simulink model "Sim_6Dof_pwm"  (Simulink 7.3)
settings: Solver=ode4  StartTime=0.0  StopTime=80  FixedStep=0.0005  MaxStep=0.0005  RelTol=1e-3
InitFcn:
  | run
StartFcn:
  | run
StopFcn:
  | Pl
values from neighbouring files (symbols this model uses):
  calfa = cos(alfa0*d2r)    [run.m]
  d2r = pi/180    (= 0.0174532925199)    [run.m]
  Kfilt = (wd1^2*wd2^2*wd3^2*wd4^2*wd5^2*wd6^2)/(wn1^2*wn2^2*wn3^2*wn4^2*wn5^2*wn6^2)    (= 0.818930549142)    [run.m]
  klr = lqr(Ap4,Bp4,Q,R)    [run.m]
  kls = lqr(Ap3,Bp3,Q,R)    [run.m]
  r2d = 180/pi    (= 57.2957795131)    [Pl.m]    (also in run.m)
  salfa = sin(alfa0*d2r)    [run.m]
  Thet0 = 43    [run.m]
  V0 = 18640    [run.m]
  wd1 = 29    [run.m]
  wd2 = 37    [run.m]
  wd3 = 40    [run.m]
  wd4 = 48    [run.m]
  wd5 = 63    [run.m]
  wd6 = 68    [run.m]
  wd7 = 34    [run.m]
  wd8 = 19.1    [run.m]
  wlp = 6.6    [run.m]
  wlp2 = 12    [run.m]
  wlpr = 12    [run.m]
  wn1 = 30    [run.m]
  wn2 = 37.9    [run.m]
  wn3 = 40.2    [run.m]
  wn4 = 48.6    [run.m]
  wn5 = 64    [run.m]
  wn6 = 68.6    [run.m]
  wn7 = 34    [run.m]
  wn8 = 19.1    [run.m]
  zd1 = 0.12    [run.m]
  zd2 = 0.12    [run.m]
  zd3 = 0.1    [run.m]
  zd4 = 0.1    [run.m]
  zd5 = 0.1    [run.m]
  zd6 = 0.1    [run.m]
  zd7 = 0.1    [run.m]
  zd8 = 0.1    [run.m]
  zlp = 0.9    [run.m]
  zlp2 = 0.7    [run.m]
  zlpr = 0.7    [run.m]
  zn1 = 0.008    [run.m]
  zn2 = 0.01    [run.m]
  zn3 = 0.01    [run.m]
  zn4 = 0.02    [run.m]
  zn5 = 0.01    [run.m]
  zn6 = 0.01    [run.m]
  zn7 = 0.01    [run.m]
  zn8 = 0.01    [run.m]
undefined symbols (not defined in the file or in its folder): Aai, Aao, Af, Bai, Bao, Bf, Cai, Cao, Cf, Dai, Dao, Df, KSmix, Pos_Thrust3
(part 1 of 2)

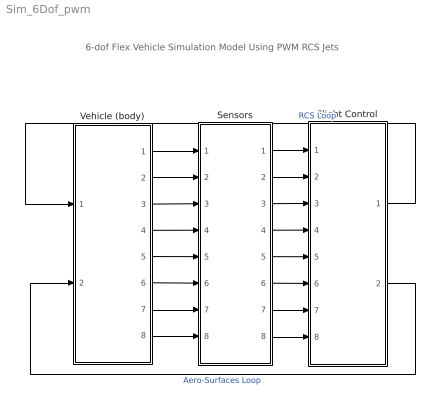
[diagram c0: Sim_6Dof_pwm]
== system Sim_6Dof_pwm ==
  note: 6-dof Flex Vehicle Simulation Model Using PWM RCS Jets
  Flight Control : Subsystem
  Sensors : Subsystem
  Vehicle (body) : Subsystem
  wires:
  Flight Control/2(Aer_pqr) -> Vehicle (body)/2(Aer_pqr)  "Aero-Surfaces Loop"
  Sensors/1(phio) -> Flight Control/1(phi)
  Sensors/2(pbo) -> Flight Control/2(pb)
  Sensors/3(rbo) -> Flight Control/3(rb)
  Sensors/4(beto) -> Flight Control/4(beta)
  Sensors/5(theto) -> Flight Control/5(thet)
  Sensors/6(qo) -> Flight Control/6(q)
  Sensors/7(alfo) -> Flight Control/7(alfa)
  Sensors/8(Nzo) -> Flight Control/8(Nz)
  Vehicle (body)/1(phi) -> Sensors/1(phi)
  Vehicle (body)/2(p) -> Sensors/2(pb)
  Vehicle (body)/3(r) -> Sensors/3(rb)
  Vehicle (body)/4(bet) -> Sensors/4(beta)
  Vehicle (body)/5(thet) -> Sensors/5(thet)
  Vehicle (body)/6(q) -> Sensors/6(q)
  Vehicle (body)/7(alf) -> Sensors/7(alfa)
  Vehicle (body)/8(Nz) -> Sensors/8(Nz)
  Flight Control/1(Jet_pqr) -> Vehicle (body)/1(Jet_PQR_Nz)  "RCS Loop"

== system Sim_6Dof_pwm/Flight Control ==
  note: Flight Control System
  phi : Inport  OutDataType=sfix(16)  OutScaling=2^0
  pb : Inport  Port=2  OutDataType=sfix(16)  OutScaling=2^0
  rb : Inport  Port=3  OutDataType=sfix(16)  OutScaling=2^0
  beta : Inport  Port=4  OutDataType=sfix(16)  OutScaling=2^0
  thet : Inport  Port=5  OutDataType=sfix(16)  OutScaling=2^0
  q : Inport  Port=6  OutDataType=sfix(16)  OutScaling=2^0
  alfa : Inport  Port=7  OutDataType=sfix(16)  OutScaling=2^0
  Nz : Inport  Port=8  OutDataType=sfix(16)  OutScaling=2^0
  1 deg  alfa-comd : Constant  Value=1*d2r  OutDataType=sfix(16)  OutScaling=2^0
  40 deg  phi-cmd : Constant  Value=40*d2r  OutDataType=sfix(16)  OutScaling=2^0
  Body 2 Stabil Transform : Subsystem
  Lateral  Flight Control : Subsystem
  Mix : Subsystem
  Mux1 : Mux  Inputs=[3,1]
  Pitch Flight Control : Subsystem
  Jet_pqr : Outport  OutDataType=sfix(16)  OutScaling=2^0
  Aer_pqr : Outport  Port=2  OutDataType=sfix(16)  OutScaling=2^0
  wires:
  Mux1/1 -> Jet_pqr/1
  Pitch Flight Control/3(Nzfb) -> Mux1/2
  40 deg  phi-cmd/1 -> Lateral  Flight Control/4(phi-cmd)
  1 deg  alfa-comd/1 -> Pitch Flight Control/5(alf-cmd)
  Mix/1(Jet_pqr) -> Mux1/1  "3"
  Nz/1 -> Pitch Flight Control/4(Nz)
  phi/1 -> Body 2 Stabil Transform/1(phi)
  pb/1 -> Body 2 Stabil Transform/2(p_b)
  rb/1 -> Body 2 Stabil Transform/3(r_b)
  Body 2 Stabil Transform/1(p_s) -> Lateral  Flight Control/1(ps)
  Body 2 Stabil Transform/2(r_s) -> Lateral  Flight Control/2(rs)
  alfa/1 -> Pitch Flight Control/3(alf)
  q/1 -> Pitch Flight Control/2(q)
  thet/1 -> Pitch Flight Control/1(thet)
  Mix/2(Aer_pqr) -> Aer_pqr/1  "3"
  beta/1 -> Lateral  Flight Control/3(beta)
  Pitch Flight Control/2(aero_Q) -> Mix/4(Aer_Q)
  Pitch Flight Control/1(rcs_Q) -> Mix/3(Rcs_Q)
  Lateral  Flight Control/2(Aero_PR) -> Mix/2(Aer_PR)
  Lateral  Flight Control/1(Rcs_PR) -> Mix/1(Rcs_PR)

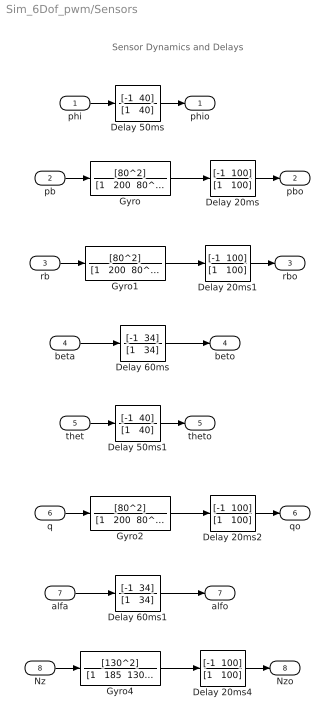
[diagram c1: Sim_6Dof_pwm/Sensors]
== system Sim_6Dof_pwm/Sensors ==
  note: Sensor Dynamics and Delays
  phi : Inport  OutDataType=sfix(16)  OutScaling=2^0
  pb : Inport  Port=2  OutDataType=sfix(16)  OutScaling=2^0
  rb : Inport  Port=3  OutDataType=sfix(16)  OutScaling=2^0
  beta : Inport  Port=4  OutDataType=sfix(16)  OutScaling=2^0
  thet : Inport  Port=5  OutDataType=sfix(16)  OutScaling=2^0
  q : Inport  Port=6  OutDataType=sfix(16)  OutScaling=2^0
  alfa : Inport  Port=7  OutDataType=sfix(16)  OutScaling=2^0
  Nz : Inport  Port=8  OutDataType=sfix(16)  OutScaling=2^0
  Delay 20ms{,1..2,4} (4 alike) : TransferFcn  Numerator="[-1  100]"  Denominator="[1   100]"
  Delay 50ms : TransferFcn  Numerator="[-1  40]"  Denominator="[1   40]"
  Delay 50ms1 : TransferFcn  Numerator="[-1  40]"  Denominator="[1   40]"
  Delay 60ms : TransferFcn  Numerator="[-1  34]"  Denominator="[1   34]"
  Delay 60ms1 : TransferFcn  Numerator="[-1  34]"  Denominator="[1   34]"
  Gyro : TransferFcn  Numerator=[80^2]  Denominator="[1   200  80^2]"
  Gyro1 : TransferFcn  Numerator=[80^2]  Denominator="[1   200  80^2]"
  Gyro2 : TransferFcn  Numerator=[80^2]  Denominator="[1   200  80^2]"
  Gyro4 : TransferFcn  Numerator=[130^2]  Denominator="[1   185  130^2]"
  phio : Outport  OutDataType=sfix(16)  OutScaling=2^0
  pbo : Outport  Port=2  OutDataType=sfix(16)  OutScaling=2^0
  rbo : Outport  Port=3  OutDataType=sfix(16)  OutScaling=2^0
  beto : Outport  Port=4  OutDataType=sfix(16)  OutScaling=2^0
  theto : Outport  Port=5  OutDataType=sfix(16)  OutScaling=2^0
  qo : Outport  Port=6  OutDataType=sfix(16)  OutScaling=2^0
  alfo : Outport  Port=7  OutDataType=sfix(16)  OutScaling=2^0
  Nzo : Outport  Port=8  OutDataType=sfix(16)  OutScaling=2^0
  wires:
  Nz/1 -> Gyro4/1
  Delay 20ms4/1 -> Nzo/1
  Gyro4/1 -> Delay 20ms4/1
  Delay 60ms1/1 -> alfo/1
  alfa/1 -> Delay 60ms1/1
  q/1 -> Gyro2/1
  Delay 20ms2/1 -> qo/1
  Gyro2/1 -> Delay 20ms2/1
  Delay 50ms1/1 -> theto/1
  thet/1 -> Delay 50ms1/1
  Delay 60ms/1 -> beto/1
  beta/1 -> Delay 60ms/1
  rb/1 -> Gyro1/1
  Delay 20ms1/1 -> rbo/1
  Gyro1/1 -> Delay 20ms1/1
  pb/1 -> Gyro/1
  Delay 20ms/1 -> pbo/1
  Delay 50ms/1 -> phio/1
  phi/1 -> Delay 50ms/1
  Gyro/1 -> Delay 20ms/1

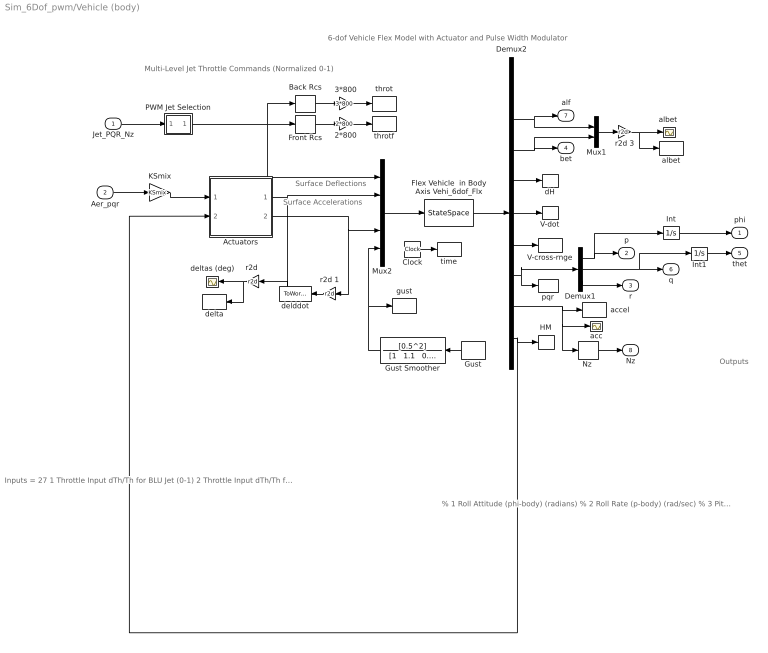
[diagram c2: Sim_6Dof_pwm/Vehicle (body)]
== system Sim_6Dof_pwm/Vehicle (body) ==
  note: Inputs = 27 1 Throttle Input dTh/Th for BLU Jet (0-1) 2 Throttle Input dTh/Th for BRU Jet (0-1) 3 Throttle Input dTh/Th for BLD Jet (0-1) 4 Throttle Input dTh/Th for BRD Jet (0-1) 5 Throttle Input dTh/Th for BL+Y Jet (0-1) 6 Throttle Input dTh/Th for BR-Y Jet (0-1) 7 Throttle Input dTh/Th for FU Jet (0-1) 8 Throttle Input dTh/Th for FLD Jet (0-1) 9 Throttle Input dTh/Th for FRD Jet (0-1) 10 Throttle Input dTh/Th for FL+Y Jet (0-1) 11 Throttle Input dTh/Th for FR-Y Jet (0-1) 12 Left Outbrd Elevon Deflection (radians) 13 Left Inboard Elevon Deflection (radians) 14 Right Inbrd Elevon Deflection (radians) 15 Right Outbrd Elevon Deflection (radians) 16 Vertical Rudder Deflection (radians) 17 Left Outbrd Elevon Velocity (rad/sec) 18 Left Inboard Elevon Velocity (rad/sec) 19 Right Inbrd Elevon Velocity (rad/sec) 20 Right Outbrd Elevon Velocity (rad/sec) 21 Vertical Rudder Velocity (rad/sec) 22 Left Outbrd Elevon Acceleration (rad/s^2) 23 Left Inboard Elevon Acceleration (rad/s^2) 24 Right Inbrd Elevon Acceleration (rad/s^2) 25 Right Outbrd Elevon Acceleration (rad/s^2) 26 Vertical Rudder Acceleration (rad/s^2) 27 Gust Veloc. Azim,Elev=(45, 90) (deg)
  note: Surface Accelerations
  note: Outputs
  note: 6-dof Vehicle Flex Model with Actuator and Pulse Width Modulator
  note: % 1 Roll Attitude (phi-body) (radians) % 2 Roll Rate (p-body) (rad/sec) % 3 Pitch Attitude (thet-bdy) (radians) % 4 Pitch Rate (q-body) (rad/sec) % 5 Yaw Attitude (psi-body) (radians) % 6 Yaw Rate (r-body) (rad/sec) % 7 Angle of attack, alfa, (radians) % 8 Angle of sideslip, beta, (radian) % 9 Change in Altitude, delta-h, (feet) % 10 Forward Acceleration (V-dot) (ft/sec) % 11 Cross Range Velocity (Vcr) (ft/sec) % 12 Rate-Gyro # 1, Roll Rate (Body) (rad/sec) % 13 Rate-Gyro # 2, Pitch Rate (Body) (rad/sec) % 14 Rate-Gyro # 3, Yaw Rate (Body) (rad/sec) % 15 Accelerom # 1, (along X), (ft/sec^2) Translat. Acceler % 16 Accelerom # 2, (along Y), (ft/sec^2) Translat. Acceler % 17 Accelerom # 3, (along Z), (ft/sec^2) Translat. Acceler % 18 Hinge Moment for Aero Surface # 1, (ft-lb) % 19 Hinge Moment for Aero Surface # 2, (ft-lb) % 20 Hinge Moment for Aero Surface # 3, (ft-lb) % 21 Hinge Moment for Aero Surface # 4, (ft-lb) % 22 Hinge Moment for Aero Surface # 5, (ft-lb)
  note: Multi-Level Jet Throttle Commands (Normalized 0-1)
  note: Surface Deflections
  Jet_PQR_Nz : Inport  OutDataType=sfix(16)  OutScaling=2^0
  Aer_pqr : Inport  Port=2  OutDataType=sfix(16)  OutScaling=2^0
  2*800 : Gain  Gain=2*800  ParameterDataType=sfix(16)  ParameterScaling=2^0  OutDataType=sfix(16)  OutScaling=2^0
  3*800 : Gain  Gain=3*800  ParameterDataType=sfix(16)  ParameterScaling=2^0  OutDataType=sfix(16)  OutScaling=2^0
  Actuators : Subsystem
  Back Rcs : Selector  InputPortWidth=11  IndexOptions=Index vector (dialog)  Indices=[1:6]  OutputSizes=1
  Clock : Clock
  Demux1 : Demux  Outputs=3
  Demux2 : Demux  Outputs="[6 1 1 1 1 1 3  3  5]"
  Flex Vehicle  in Body Axis Vehi_6dof_Flx : StateSpace  A=Af  B=Bf  C=Cf  D=Df
  Front Rcs : Selector  InputPortWidth=11  IndexOptions=Index vector (dialog)  Indices=[7:11]  OutputSizes=1
  Gust : DiscretePulseGenerator  PulseType=Time based  Amplitude=50  Period=500  PulseWidth=10  PhaseDelay=0  SampleTime=1
  Gust Smoother : TransferFcn  Numerator=[0.5^2]  Denominator="[1   1.1   0.5^2]"
  HM : ToWorkspace  VariableName=HM  SampleTime=-1  SaveFormat=Array
  Int : Integrator
  Int1 : Integrator
  KSmix : Gain  Gain=KSmix  Multiplication=Matrix(K*u)  ParameterDataType=sfix(16)  ParameterScaling=2^0  OutDataType=sfix(16)  OutScaling=2^0
  Mux1 : Mux  Inputs=2
  Mux2 : Mux  Inputs=[11, 5,5,5, 1]
  "Nz " : Selector  InputPortWidth=3  IndexOptions=Index vector (dialog)  Indices=[3]  OutputSizes=1
  PWM Jet Selection : Subsystem
  V-cross-rnge : ToWorkspace  VariableName=Vxrng  SampleTime=-1  SaveFormat=Array
  V-dot : ToWorkspace  VariableName=dV  SampleTime=-1  SaveFormat=Array
  acc : Scope
  accel : ToWorkspace  VariableName=accel  SampleTime=-1  SaveFormat=Array
  albet : ToWorkspace  VariableName=albet  SampleTime=-1  SaveFormat=Array
  "albet " : Scope
  dH : ToWorkspace  VariableName=dH  SampleTime=-1  SaveFormat=Array
  delddot : ToWorkspace  VariableName=delddot  SampleTime=-1  SaveFormat=Array
  delta : ToWorkspace  VariableName=delta  SampleTime=-1  SaveFormat=Array
  deltas (deg) : Scope
  gust : ToWorkspace  VariableName=gust  SampleTime=-1  SaveFormat=Array
  pqr : ToWorkspace  VariableName=pqr  SampleTime=-1  SaveFormat=Array
  "r2d " : Gain  Gain=r2d  ParameterDataType=sfix(16)  ParameterScaling=2^0  OutDataType=sfix(16)  OutScaling=2^0
  r2d 1 : Gain  Gain=r2d  ParameterDataType=sfix(16)  ParameterScaling=2^0  OutDataType=sfix(16)  OutScaling=2^0
  r2d 3 : Gain  Gain=r2d  ParameterDataType=sfix(16)  ParameterScaling=2^0  OutDataType=sfix(16)  OutScaling=2^0
  throt : ToWorkspace  VariableName=throtb  SampleTime=-1  SaveFormat=Array
  throtf : ToWorkspace  VariableName=throtf  SampleTime=-1  SaveFormat=Array
  time : ToWorkspace  VariableName=time  SampleTime=-1  SaveFormat=Array
  phi : Outport  OutDataType=sfix(16)  OutScaling=2^0
  p : Outport  Port=2  OutDataType=sfix(16)  OutScaling=2^0
  r : Outport  Port=3  OutDataType=sfix(16)  OutScaling=2^0
  bet : Outport  Port=4  OutDataType=sfix(16)  OutScaling=2^0
  thet : Outport  Port=5  OutDataType=sfix(16)  OutScaling=2^0
  q : Outport  Port=6  OutDataType=sfix(16)  OutScaling=2^0
  alf : Outport  Port=7  OutDataType=sfix(16)  OutScaling=2^0
  Nz : Outport  Port=8  OutDataType=sfix(16)  OutScaling=2^0
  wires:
  Actuators/2(delddot) -> Mux2/4, r2d 1/1
  KSmix/1 -> Actuators/1(delcom)
  Actuators/1(delta) -> Mux2/2, "r2d "/1
  Jet_PQR_Nz/1 -> PWM Jet Selection/1(In)
  Aer_pqr/1 -> KSmix/1
  Mux2/1 -> Flex Vehicle  in Body Axis Vehi_6dof_Flx/1
  PWM Jet Selection/1(Ot) -> Mux2/1, Back Rcs/1, Front Rcs/1
  "r2d "/1 -> deltas (deg)/1, delta/1
  r2d 1/1 -> delddot/1
  Gust/1 -> Gust Smoother/1
  Clock/1 -> time/1
  Gust Smoother/1 -> Mux2/5, gust/1
  r2d 3/1 -> "albet "/1, albet/1
  Mux1/1 -> r2d 3/1
  Flex Vehicle  in Body Axis Vehi_6dof_Flx/1 -> Demux2/1
  Demux2/9 -> HM/1, Actuators/2(HM)
  Demux2/8 -> accel/1, acc/1, "Nz "/1
  "Nz "/1 -> Nz/1
  Demux2/7 -> pqr/1, Demux1/1
  Demux1/1 -> p/1, Int/1
  Demux1/2 -> q/1, Int1/1
  Demux1/3 -> r/1
  Demux2/6 -> V-cross-rnge/1
  Demux2/5 -> V-dot/1
  Demux2/4 -> dH/1
  Demux2/2 -> alf/1, Mux1/1
  Demux2/3 -> bet/1, Mux1/2
  Int1/1 -> thet/1
  Int/1 -> phi/1
  Back Rcs/1 -> 3*800/1
  Front Rcs/1 -> 2*800/1
  3*800/1 -> throt/1
  2*800/1 -> throtf/1

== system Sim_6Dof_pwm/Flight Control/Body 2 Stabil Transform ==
  note: Body to Stability Axes Transformation
  phi : Inport  OutDataType=sfix(16)  OutScaling=2^0
  p_b : Inport  Port=2  OutDataType=sfix(16)  OutScaling=2^0
  r_b : Inport  Port=3  OutDataType=sfix(16)  OutScaling=2^0
  Mux1 : Mux  Inputs=2
  Sum1 : Sum  Inputs=+|+  OutDataType=sfix(16)  OutScaling=2^0
  Sum2 : Sum  Inputs=+|-  OutDataType=sfix(16)  OutScaling=2^0
  Sum3 : Sum  Inputs=|++  OutDataType=sfix(16)  OutScaling=2^0
  Sum4 : Sum  Inputs=|+-  OutDataType=sfix(16)  OutScaling=2^0
  calfa : Gain  Gain=calfa  ParameterDataType=sfix(16)  ParameterScaling=2^0  OutDataType=sfix(16)  OutScaling=2^0
  "calfa " : Gain  Gain=calfa  ParameterDataType=sfix(16)  ParameterScaling=2^0  OutDataType=sfix(16)  OutScaling=2^0
  g cos(Thet0) /V0 : Gain  Gain=32.2*cos(Thet0*d2r)/V0  ParameterDataType=sfix(16)  ParameterScaling=2^0  OutDataType=sfix(16)  OutScaling=2^0
  g sin(Thet0) /V0 : Gain  Gain=32.2*sin(Thet0*d2r)/V0  ParameterDataType=sfix(16)  ParameterScaling=2^0  OutDataType=sfix(16)  OutScaling=2^0
  pr_stabil : ToWorkspace  VariableName=pr_st  SampleTime=-1  SaveFormat=Array
  salfa : Gain  Gain=salfa  ParameterDataType=sfix(16)  ParameterScaling=2^0  OutDataType=sfix(16)  OutScaling=2^0
  "salfa " : Gain  Gain=salfa  ParameterDataType=sfix(16)  ParameterScaling=2^0  OutDataType=sfix(16)  OutScaling=2^0
  p_s : Outport  OutDataType=sfix(16)  OutScaling=2^0
  r_s : Outport  Port=2  OutDataType=sfix(16)  OutScaling=2^0
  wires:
  Mux1/1 -> pr_stabil/1
  "salfa "/1 -> Sum2/2
  "calfa "/1 -> Sum2/1
  salfa/1 -> Sum1/2
  calfa/1 -> Sum1/1
  Sum3/1 -> calfa/1, "salfa "/1
  Sum4/1 -> salfa/1, "calfa "/1
  phi/1 -> g sin(Thet0) /V0/1, g cos(Thet0) /V0/1
  g sin(Thet0) /V0/1 -> Sum4/2
  g cos(Thet0) /V0/1 -> Sum3/2
  r_b/1 -> Sum4/1
  p_b/1 -> Sum3/1
  Sum2/1 -> Mux1/2, r_s/1
  Sum1/1 -> Mux1/1, p_s/1

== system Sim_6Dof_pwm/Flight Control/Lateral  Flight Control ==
  note: Lateral Flight Control System
  ps : Inport  OutDataType=sfix(16)  OutScaling=2^0
  rs : Inport  Port=2  OutDataType=sfix(16)  OutScaling=2^0
  beta : Inport  Port=3  OutDataType=sfix(16)  OutScaling=2^0
  phi-cmd : Inport  Port=4  OutDataType=sfix(16)  OutScaling=2^0
  5 state Aero feedback : Gain  Gain=-kls  Multiplication=Matrix(K*u)  ParameterDataType=sfix(16)  ParameterScaling=2^0  OutDataType=sfix(16)  OutScaling=2^0
  5 state RCS feedback : Gain  Gain=-klr  Multiplication=Matrix(K*u)  ParameterDataType=sfix(16)  ParameterScaling=2^0  OutDataType=sfix(16)  OutScaling=2^0
  Filters : Subsystem
  Int : Integrator
  "Int " : Integrator
  Mux3 : Mux  Inputs=5
  RCS Filters : Subsystem
  Sum : Sum  Inputs=|+-  OutDataType=sfix(16)  OutScaling=2^0
  phi : Scope
  phi-stabil : ToWorkspace  VariableName=phi_st  SampleTime=-1  SaveFormat=Array
  r2d : Gain  Gain=r2d  ParameterDataType=sfix(16)  ParameterScaling=2^0  OutDataType=sfix(16)  OutScaling=2^0
  Rcs_PR : Outport  OutDataType=sfix(16)  OutScaling=2^0
  Aero_PR : Outport  Port=2  OutDataType=sfix(16)  OutScaling=2^0
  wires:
  RCS Filters/1(Ou) -> Rcs_PR/1
  Filters/1(Ou) -> Aero_PR/1
  r2d/1 -> phi-stabil/1, phi/1
  phi-cmd/1 -> Sum/2
  5 state Aero feedback/1 -> Filters/1(In)  "aero(P,R)"
  5 state RCS feedback/1 -> RCS Filters/1(In)  "rcs(P,R)"
  rs/1 -> Mux3/2
  Mux3/1 -> 5 state RCS feedback/1, 5 state Aero feedback/1
  ps/1 -> Mux3/1, "Int "/1
  beta/1 -> Mux3/3, Int/1
  Int/1 -> Mux3/5  "beti"
  Sum/1 -> Mux3/4
  "Int "/1 -> r2d/1, Sum/1  "pint"

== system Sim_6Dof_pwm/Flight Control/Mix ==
  Rcs_PR : Inport  OutDataType=sfix(16)  OutScaling=2^0
  Aer_PR : Inport  Port=2  OutDataType=sfix(16)  OutScaling=2^0
  Rcs_Q : Inport  Port=3  OutDataType=sfix(16)  OutScaling=2^0
  Aer_Q : Inport  Port=4  OutDataType=sfix(16)  OutScaling=2^0
  Demux1 : Demux  Outputs=2
  Demux2 : Demux  Outputs=2
  Mux1 : Mux  Inputs=3
  Mux2 : Mux  Inputs=3
  Jet_pqr : Outport  OutDataType=sfix(16)  OutScaling=2^0
  Aer_pqr : Outport  Port=2  OutDataType=sfix(16)  OutScaling=2^0
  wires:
  Rcs_Q/1 -> Mux1/2
  Mux2/1 -> Aer_pqr/1
  Aer_Q/1 -> Mux2/2
  Aer_PR/1 -> Demux2/1
  Rcs_PR/1 -> Demux1/1
  Mux1/1 -> Jet_pqr/1
  Demux2/2 -> Mux2/3
  Demux2/1 -> Mux2/1
  Demux1/2 -> Mux1/3
  Demux1/1 -> Mux1/1

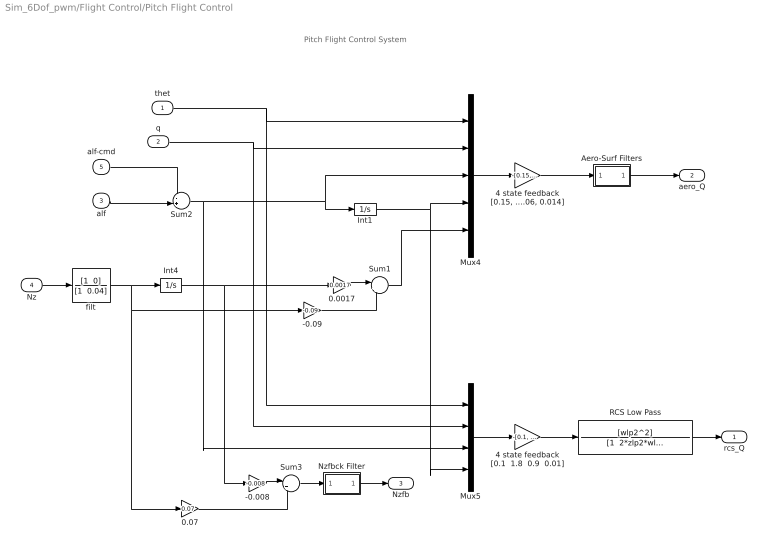
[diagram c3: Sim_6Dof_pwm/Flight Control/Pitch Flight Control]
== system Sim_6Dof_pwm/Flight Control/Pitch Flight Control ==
  note: Pitch Flight Control System
  thet : Inport  OutDataType=sfix(16)  OutScaling=2^0
  q : Inport  Port=2  OutDataType=sfix(16)  OutScaling=2^0
  alf : Inport  Port=3  OutDataType=sfix(16)  OutScaling=2^0
  Nz : Inport  Port=4  OutDataType=sfix(16)  OutScaling=2^0
  alf-cmd : Inport  Port=5  OutDataType=sfix(16)  OutScaling=2^0
  -0.008 : Gain  Gain=-0.008  ParameterDataType=sfix(16)  ParameterScaling=2^0  OutDataType=sfix(16)  OutScaling=2^0
  -0.09 : Gain  Gain=-0.09  ParameterDataType=sfix(16)  ParameterScaling=2^0  OutDataType=sfix(16)  OutScaling=2^0
  0.0017 : Gain  Gain=0.0017  ParameterDataType=sfix(16)  ParameterScaling=2^0  OutDataType=sfix(16)  OutScaling=2^0
  0.07 : Gain  Gain=0.07  ParameterDataType=sfix(16)  ParameterScaling=2^0  OutDataType=sfix(16)  OutScaling=2^0
  4 state feedback [0.1  1.8  0.9  0.01] : Gain  Gain="-[0.1,   1.8,   0.9,    0.01]"  Multiplication=Matrix(K*u)  ParameterDataType=sfix(16)  ParameterScaling=2^0  OutDataType=sfix(16)  OutScaling=2^0
  "4 state feedback [0.15, 2, 0.9, 0.06, 0.014]" : Gain  Gain="-[0.15,   2,   0.9,    0.06,   0.015]"  Multiplication=Matrix(K*u)  ParameterDataType=sfix(16)  ParameterScaling=2^0  OutDataType=sfix(16)  OutScaling=2^0
  Aero-Surf Filters : Subsystem
  Int1 : Integrator
  Int4 : Integrator
  Mux4 : Mux  Inputs=5
  Mux5 : Mux
  Nzfbck Filter : Subsystem
  RCS Low Pass : TransferFcn  Numerator=[wlp2^2]  Denominator="[1  2*zlp2*wlp2  wlp2^2]"
  Sum1 : Sum  Inputs=|++  OutDataType=sfix(16)  OutScaling=2^0
  Sum2 : Sum  Inputs=-+|  OutDataType=sfix(16)  OutScaling=2^0
  Sum3 : Sum  Inputs=|++  OutDataType=sfix(16)  OutScaling=2^0
  filt : TransferFcn  Numerator="[1  0]"  Denominator="[1  0.04]"
  rcs_Q : Outport  OutDataType=sfix(16)  OutScaling=2^0
  aero_Q : Outport  Port=2  OutDataType=sfix(16)  OutScaling=2^0
  Nzfb : Outport  Port=3  OutDataType=sfix(16)  OutScaling=2^0
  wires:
  RCS Low Pass/1 -> rcs_Q/1
  Sum3/1 -> Nzfbck Filter/1(in)
  Int1/1 -> Mux4/4, Mux5/4
  Sum2/1 -> Int1/1, Mux4/3, Mux5/3
  thet/1 -> Mux4/1, Mux5/1
  q/1 -> Mux4/2, Mux5/2
  0.0017/1 -> Sum1/1
  -0.09/1 -> Sum1/2
  Nz/1 -> filt/1
  Sum1/1 -> Mux4/5
  Mux4/1 -> "4 state feedback [0.15, 2, 0.9, 0.06, 0.014]"/1
  "4 state feedback [0.15, 2, 0.9, 0.06, 0.014]"/1 -> Aero-Surf Filters/1(in)
  Mux5/1 -> 4 state feedback [0.1  1.8  0.9  0.01]/1
  4 state feedback [0.1  1.8  0.9  0.01]/1 -> RCS Low Pass/1
  0.07/1 -> Sum3/2
  -0.008/1 -> Sum3/1
  Int4/1 -> 0.0017/1, -0.008/1
  filt/1 -> Int4/1, -0.09/1, 0.07/1
  alf/1 -> Sum2/2
  alf-cmd/1 -> Sum2/1
  Nzfbck Filter/1(ot) -> Nzfb/1
  Aero-Surf Filters/1(ot) -> aero_Q/1

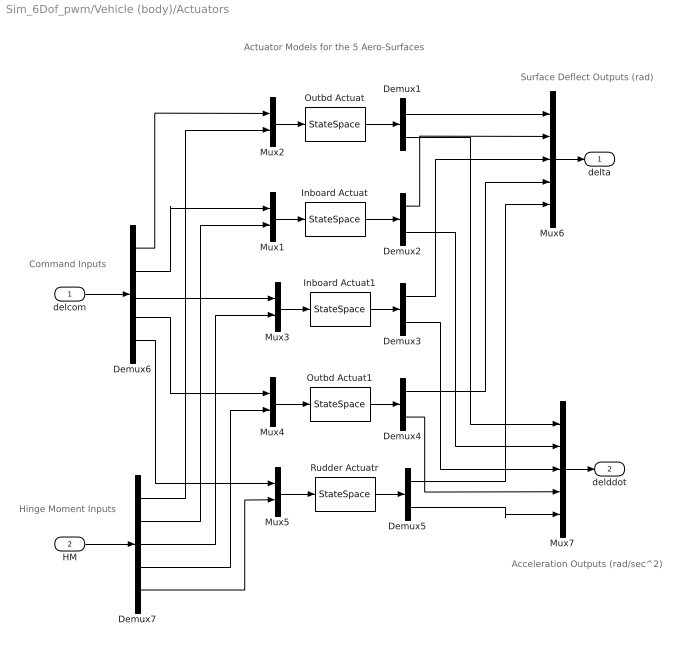
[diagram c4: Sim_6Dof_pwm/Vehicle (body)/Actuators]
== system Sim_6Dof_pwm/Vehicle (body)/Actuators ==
  note: Command Inputs
  note: Hinge Moment Inputs
  note: Actuator Models for the 5 Aero-Surfaces
  note: Acceleration Outputs (rad/sec^2)
  note: Surface Deflect Outputs (rad)
  delcom : Inport  OutDataType=sfix(16)  OutScaling=2^0
  HM : Inport  Port=2  OutDataType=sfix(16)  OutScaling=2^0
  Demux{1..5} (5 alike) : Demux  Outputs=3
  Demux6 : Demux  Outputs=5
  Demux7 : Demux  Outputs=5
  Inboard Actuat : StateSpace  A=Aai  B=Bai  C=Cai  D=Dai
  Inboard Actuat1 : StateSpace  A=Aai  B=Bai  C=Cai  D=Dai
  Mux{1..5} (5 alike) : Mux  Inputs=2
  Mux6 : Mux  Inputs=5
  Mux7 : Mux  Inputs=5
  Outbd Actuat : StateSpace  A=Aao  B=Bao  C=Cao  D=Dao
  Outbd Actuat1 : StateSpace  A=Aao  B=Bao  C=Cao  D=Dao
  Rudder Actuatr : StateSpace  A=Aai  B=Bai  C=Cai  D=Dai
  delta : Outport  OutDataType=sfix(16)  OutScaling=2^0
  delddot : Outport  Port=2  OutDataType=sfix(16)  OutScaling=2^0
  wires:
  Mux6/1 -> delta/1
  Mux7/1 -> delddot/1
  Mux1/1 -> Inboard Actuat/1
  Mux2/1 -> Outbd Actuat/1
  Mux3/1 -> Inboard Actuat1/1
  Mux4/1 -> Outbd Actuat1/1
  Mux5/1 -> Rudder Actuatr/1
  Outbd Actuat/1 -> Demux1/1
  Inboard Actuat/1 -> Demux2/1
  Inboard Actuat1/1 -> Demux3/1
  Outbd Actuat1/1 -> Demux4/1
  Rudder Actuatr/1 -> Demux5/1
  delcom/1 -> Demux6/1
  Demux6/1 -> Mux2/1
  Demux6/2 -> Mux1/1
  Demux6/3 -> Mux3/1
  Demux6/4 -> Mux4/1
  Demux6/5 -> Mux5/1
  Demux5/3 -> Mux7/5
  Demux4/3 -> Mux7/4
  Demux3/3 -> Mux7/3
  Demux2/3 -> Mux7/2
  Demux1/3 -> Mux7/1
  Demux1/1 -> Mux6/1
  Demux2/1 -> Mux6/2
  Demux3/1 -> Mux6/3
  Demux4/1 -> Mux6/4
  Demux5/1 -> Mux6/5
  Demux7/1 -> Mux2/2
  Demux7/2 -> Mux1/2
  Demux7/3 -> Mux3/2
  Demux7/4 -> Mux4/2
  Demux7/5 -> Mux5/2
  HM/1 -> Demux7/1

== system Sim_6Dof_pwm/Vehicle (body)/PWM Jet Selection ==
  note: Jet Selection Logic
  In : Inport  OutDataType=sfix(16)  OutScaling=2^0
  Demux2 : Demux  Outputs="[3  3  3  3  3  3  2  2  2  2  2  1]"
  Mem : Memory
  Mix Logic +ve thrusts : MATLABFcn  MATLABFcn=Pos_Thrust3(u(1:4) )  OutputDimensions=6*3 + 5*2 + 1  OutputSignalType=real
  Mux1 : Mux  Inputs=11
  PW Modulators : Subsystem
  error : Scope
  error-magn : ToWorkspace  VariableName=erm  SampleTime=-1  SaveFormat=Array
  Ot : Outport  OutDataType=sfix(16)  OutScaling=2^0
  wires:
  Demux2/12 -> error-magn/1, error/1
  Mix Logic +ve thrusts/1 -> Demux2/1
  PW Modulators/11(O10) -> Mux1/11
  PW Modulators/10(O9) -> Mux1/10
  PW Modulators/9(O8) -> Mux1/9
  PW Modulators/8(O7) -> Mux1/8
  PW Modulators/7(O6) -> Mux1/7
  PW Modulators/6(O5) -> Mux1/6
  PW Modulators/5(O4) -> Mux1/5
  PW Modulators/4(O3) -> Mux1/4
  PW Modulators/3(O2) -> Mux1/3
  PW Modulators/2(O1) -> Mux1/2
  PW Modulators/1(O) -> Mux1/1
  Demux2/11 -> PW Modulators/11(In10)
  Demux2/10 -> PW Modulators/10(In9)
  Demux2/9 -> PW Modulators/9(In8)
  Demux2/8 -> PW Modulators/8(In7)
  Demux2/7 -> PW Modulators/7(In6)
  Demux2/6 -> PW Modulators/6(In5)
  Demux2/5 -> PW Modulators/5(In4)
  Demux2/4 -> PW Modulators/4(In3)
  Demux2/3 -> PW Modulators/3(In2)
  Demux2/2 -> PW Modulators/2(In1)
  Demux2/1 -> PW Modulators/1(In)
  Mem/1 -> Mix Logic +ve thrusts/1
  Mux1/1 -> Ot/1
  In/1 -> Mem/1

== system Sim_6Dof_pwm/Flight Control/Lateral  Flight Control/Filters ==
  In : Inport  OutDataType=sfix(16)  OutScaling=2^0
  19.1 r/s Notch1 : TransferFcn  Numerator="[1  2*zn8*wn8  wn8^2]"  Denominator="[1  2*zd8*wd8  wd8^2]"
  34 r/s Notch : TransferFcn  Numerator="[1  2*zn7*wn7  wn7^2]"  Denominator="[1  2*zd7*wd7  wd7^2]"
  Demux1 : Demux  Outputs=2
  Mux1 : Mux  Inputs=2
  Roll Low Pass : TransferFcn  Numerator=[wlp^2]  Denominator="[1  1.3*wlp  wlp^2]"
  Yaw Low Pass : TransferFcn  Numerator=[wlp^2]  Denominator="[1  1.3*wlp  wlp^2]"
  Ou : Outport  OutDataType=sfix(16)  OutScaling=2^0
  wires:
  19.1 r/s Notch1/1 -> Yaw Low Pass/1
  34 r/s Notch/1 -> Roll Low Pass/1
  Yaw Low Pass/1 -> Mux1/2
  Demux1/2 -> 19.1 r/s Notch1/1
  Roll Low Pass/1 -> Mux1/1
  Mux1/1 -> Ou/1
  Demux1/1 -> 34 r/s Notch/1
  In/1 -> Demux1/1

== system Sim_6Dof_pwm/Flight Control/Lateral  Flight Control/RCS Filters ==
  In : Inport  OutDataType=sfix(16)  OutScaling=2^0
  Demux1 : Demux  Outputs=2
  Mux1 : Mux  Inputs=2
  RCS Low Pass : TransferFcn  Numerator=[wlpr^2]  Denominator="[1  2*zlpr*wlpr  wlpr^2]"
  RCS Low Pass1 : TransferFcn  Numerator=[wlpr^2]  Denominator="[1  2*zlpr*wlpr  wlpr^2]"
  Ou : Outport  OutDataType=sfix(16)  OutScaling=2^0
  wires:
  RCS Low Pass1/1 -> Mux1/2
  RCS Low Pass/1 -> Mux1/1
  Demux1/2 -> RCS Low Pass1/1
  Mux1/1 -> Ou/1
  Demux1/1 -> RCS Low Pass/1
  In/1 -> Demux1/1

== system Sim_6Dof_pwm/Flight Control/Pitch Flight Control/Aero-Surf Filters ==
  note: Pitch Flexibility Filters
  in : Inport  OutDataType=sfix(16)  OutScaling=2^0
  30 r/s Notch : TransferFcn  Numerator="[1  2*zn1*wn1  wn1^2]"  Denominator="[1  2*zd1*wd1  wd1^2]"
  34 r/s Notch1 : TransferFcn  Numerator="[1  2*zn7*wn7  wn7^2]"  Denominator="[1  2*zd7*wd7  wd7^2]"
  37.9 r/s Notch : TransferFcn  Numerator="[1  2*zn2*wn2  wn2^2]"  Denominator="[1  2*zd2*wd2  wd2^2]"
  40.2 r/s Notch : TransferFcn  Numerator="[1  2*zn3*wn3  wn3^2]"  Denominator="[1  2*zd3*wd3  wd3^2]"
  48.6 r/s Notch : TransferFcn  Numerator="[1  2*zn4*wn4  wn4^2]"  Denominator="[1  2*zd4*wd4  wd4^2]"
  64 r/s Notch : TransferFcn  Numerator="[1  2*zn5*wn5  wn5^2]"  Denominator="[1  2*zd5*wd5  wd5^2]"
  68 r/s Notch : TransferFcn  Numerator="[1  2*zn6*wn6  wn6^2]"  Denominator="[1  2*zd6*wd6  wd6^2]"
  9 r/s Notch : TransferFcn  Numerator="[1  0.04*9  8.5^2]"  Denominator="[1  0.2*9  8.5^2]"
  Kfilt : Gain  Gain=Kfilt  ParameterDataType=sfix(16)  ParameterScaling=2^0  OutDataType=sfix(16)  OutScaling=2^0
  Low Pass : TransferFcn  Numerator=[wlp^2]  Denominator="[1  2*zlp*wlp  wlp^2]"
  ot : Outport  OutDataType=sfix(16)  OutScaling=2^0
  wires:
  in/1 -> 30 r/s Notch/1
  30 r/s Notch/1 -> 37.9 r/s Notch/1
  37.9 r/s Notch/1 -> 40.2 r/s Notch/1
  40.2 r/s Notch/1 -> 48.6 r/s Notch/1
  Kfilt/1 -> ot/1
  68 r/s Notch/1 -> 34 r/s Notch1/1
  Low Pass/1 -> Kfilt/1
  48.6 r/s Notch/1 -> 64 r/s Notch/1
  64 r/s Notch/1 -> 68 r/s Notch/1
  9 r/s Notch/1 -> Low Pass/1
  34 r/s Notch1/1 -> 9 r/s Notch/1

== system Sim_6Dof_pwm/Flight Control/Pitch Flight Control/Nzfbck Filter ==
  note: Nz feedback Filters
  in : Inport  OutDataType=sfix(16)  OutScaling=2^0
  30 r/s Notch : TransferFcn  Numerator="[1  2*zn1*wn1  wn1^2]"  Denominator="[1  2*zd1*wd1  wd1^2]"
  RCS Low Pass1 : TransferFcn  Numerator=[wlp2^2]  Denominator="[1  2*zlp2*wlp2  wlp2^2]"
  ot : Outport  OutDataType=sfix(16)  OutScaling=2^0
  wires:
  in/1 -> 30 r/s Notch/1
  30 r/s Notch/1 -> RCS Low Pass1/1
  RCS Low Pass1/1 -> ot/1

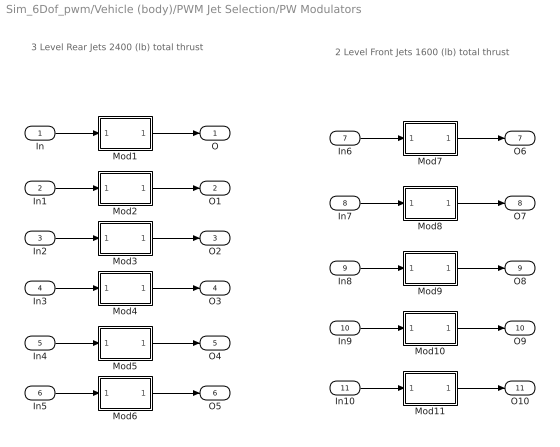
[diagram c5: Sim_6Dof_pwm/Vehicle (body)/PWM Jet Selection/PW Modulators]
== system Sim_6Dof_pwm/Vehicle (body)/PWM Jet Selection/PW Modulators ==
  note: 2 Level Front Jets 1600 (lb) total thrust
  note: 3 Level Rear Jets 2400 (lb) total thrust
  In : Inport  OutDataType=sfix(16)  OutScaling=2^0
  In1 : Inport  Port=2  OutDataType=sfix(16)  OutScaling=2^0
  In2 : Inport  Port=3  OutDataType=sfix(16)  OutScaling=2^0
  In3 : Inport  Port=4  OutDataType=sfix(16)  OutScaling=2^0
  In4 : Inport  Port=5  OutDataType=sfix(16)  OutScaling=2^0
  In5 : Inport  Port=6  OutDataType=sfix(16)  OutScaling=2^0
  In6 : Inport  Port=7  OutDataType=sfix(16)  OutScaling=2^0
  In7 : Inport  Port=8  OutDataType=sfix(16)  OutScaling=2^0
  In8 : Inport  Port=9  OutDataType=sfix(16)  OutScaling=2^0
  In9 : Inport  Port=10  OutDataType=sfix(16)  OutScaling=2^0
  In10 : Inport  Port=11  OutDataType=sfix(16)  OutScaling=2^0
  Mod1 : Subsystem
  Mod10 : Subsystem
  Mod11 : Subsystem
  Mod2 : Subsystem
  Mod3 : Subsystem
  Mod4 : Subsystem
  Mod5 : Subsystem
  Mod6 : Subsystem
  Mod7 : Subsystem
  Mod8 : Subsystem
  Mod9 : Subsystem
  O : Outport  OutDataType=sfix(16)  OutScaling=2^0
  O1 : Outport  Port=2  OutDataType=sfix(16)  OutScaling=2^0
  O2 : Outport  Port=3  OutDataType=sfix(16)  OutScaling=2^0
  O3 : Outport  Port=4  OutDataType=sfix(16)  OutScaling=2^0
  O4 : Outport  Port=5  OutDataType=sfix(16)  OutScaling=2^0
  O5 : Outport  Port=6  OutDataType=sfix(16)  OutScaling=2^0
  O6 : Outport  Port=7  OutDataType=sfix(16)  OutScaling=2^0
  O7 : Outport  Port=8  OutDataType=sfix(16)  OutScaling=2^0
  O8 : Outport  Port=9  OutDataType=sfix(16)  OutScaling=2^0
  O9 : Outport  Port=10  OutDataType=sfix(16)  OutScaling=2^0
  O10 : Outport  Port=11  OutDataType=sfix(16)  OutScaling=2^0
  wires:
  In10/1 -> Mod11/1(In1)
  Mod11/1(O1) -> O10/1
  In9/1 -> Mod10/1(In1)
  Mod10/1(O1) -> O9/1
  In8/1 -> Mod9/1(In1)
  Mod9/1(O1) -> O8/1
  In7/1 -> Mod8/1(In1)
  Mod8/1(O1) -> O7/1
  In6/1 -> Mod7/1(In1)
  Mod7/1(O1) -> O6/1
  In5/1 -> Mod6/1(In1)
  Mod6/1(O1) -> O5/1
  In4/1 -> Mod5/1(In1)
  Mod5/1(O1) -> O4/1
  In3/1 -> Mod4/1(In1)
  Mod4/1(O1) -> O3/1
  In2/1 -> Mod3/1(In1)
  Mod3/1(O1) -> O2/1
  In1/1 -> Mod2/1(In1)
  Mod2/1(O1) -> O1/1
  In/1 -> Mod1/1(In1)
  Mod1/1(O1) -> O/1

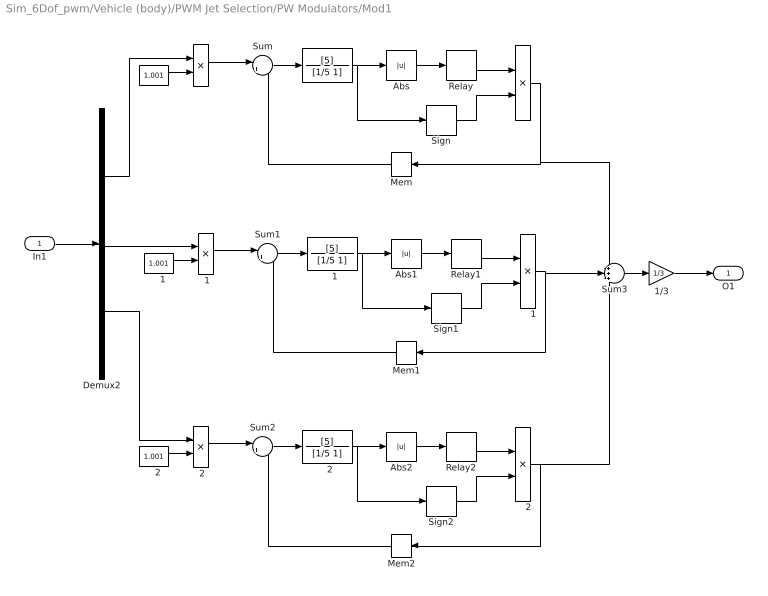
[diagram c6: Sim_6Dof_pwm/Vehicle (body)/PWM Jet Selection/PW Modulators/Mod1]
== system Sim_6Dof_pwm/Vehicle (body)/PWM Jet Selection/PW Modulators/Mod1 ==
  In1 : Inport  OutDataType=sfix(16)  OutScaling=2^0
  " " : Product  OutDataType=sfix(16)  OutScaling=2^0
  "  " : TransferFcn  Numerator=[5]  Denominator=[1/5 1]
  "   " : Constant  Value=1.001  OutDataType=sfix(16)  OutScaling=2^0
  "    " : Product  OutDataType=sfix(16)  OutScaling=2^0
  "    1" : Product  OutDataType=sfix(16)  OutScaling=2^0
  "    2" : Product  OutDataType=sfix(16)  OutScaling=2^0
  "   1" : Constant  Value=1.001  OutDataType=sfix(16)  OutScaling=2^0
  "   2" : Constant  Value=1.001  OutDataType=sfix(16)  OutScaling=2^0
  "  1" : TransferFcn  Numerator=[5]  Denominator=[1/5 1]
  "  2" : TransferFcn  Numerator=[5]  Denominator=[1/5 1]
  " 1" : Product  OutDataType=sfix(16)  OutScaling=2^0
  " 2" : Product  OutDataType=sfix(16)  OutScaling=2^0
  1/3 : Gain  Gain=1/3  ParameterDataType=sfix(16)  ParameterScaling=2^0  OutDataType=sfix(16)  OutScaling=2^0
  Abs : Abs
  Abs1 : Abs
  Abs2 : Abs
  Demux2 : Demux  Outputs=3
  Mem : Memory
  Mem1 : Memory
  Mem2 : Memory
  Relay : Relay  OnSwitchValue=0.5  OffSwitchValue=0.5  OutDataType=sfix(16)  OutScaling=2^0
  Relay1 : Relay  OnSwitchValue=0.5  OffSwitchValue=0.5  OutDataType=sfix(16)  OutScaling=2^0
  Relay2 : Relay  OnSwitchValue=0.5  OffSwitchValue=0.5  OutDataType=sfix(16)  OutScaling=2^0
  Sign : Signum
  Sign1 : Signum
  Sign2 : Signum
  Sum : Sum  Inputs=|+-  OutDataType=sfix(16)  OutScaling=2^0
  Sum1 : Sum  Inputs=|+-  OutDataType=sfix(16)  OutScaling=2^0
  Sum2 : Sum  Inputs=|+-  OutDataType=sfix(16)  OutScaling=2^0
  Sum3 : Sum  Inputs=+++  OutDataType=sfix(16)  OutScaling=2^0
  O1 : Outport  OutDataType=sfix(16)  OutScaling=2^0
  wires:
  1/3/1 -> O1/1
  Sum3/1 -> 1/3/1
  In1/1 -> Demux2/1
  Demux2/3 -> " 2"/1
  Demux2/1 -> " "/1
  Demux2/2 -> " 1"/1
  " 2"/1 -> Sum2/1
  "   2"/1 -> " 2"/2
  Sum2/1 -> "  2"/1
  "  2"/1 -> Abs2/1, Sign2/1
  Abs2/1 -> Relay2/1
  Relay2/1 -> "    2"/1
  Sign2/1 -> "    2"/2
  Mem2/1 -> Sum2/2
  "    2"/1 -> Sum3/3, Mem2/1
  " 1"/1 -> Sum1/1
  "   1"/1 -> " 1"/2
  Sum1/1 -> "  1"/1
  "  1"/1 -> Abs1/1, Sign1/1
  Abs1/1 -> Relay1/1
  Relay1/1 -> "    1"/1
  Sign1/1 -> "    1"/2
  Mem1/1 -> Sum1/2
  "    1"/1 -> Sum3/2, Mem1/1
  " "/1 -> Sum/1
  "   "/1 -> " "/2
  Sum/1 -> "  "/1
  "  "/1 -> Abs/1, Sign/1
  Abs/1 -> Relay/1
  Relay/1 -> "    "/1
  Sign/1 -> "    "/2
  Mem/1 -> Sum/2
  "    "/1 -> Sum3/1, Mem/1

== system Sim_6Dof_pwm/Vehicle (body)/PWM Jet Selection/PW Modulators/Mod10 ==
  In1 : Inport  OutDataType=sfix(16)  OutScaling=2^0
  " " : Product  OutDataType=sfix(16)  OutScaling=2^0
  "  " : TransferFcn  Numerator=[5]  Denominator=[1/5 1]
  "   " : Constant  Value=1.001  OutDataType=sfix(16)  OutScaling=2^0
  "    " : Product  OutDataType=sfix(16)  OutScaling=2^0
  "    1" : Product  OutDataType=sfix(16)  OutScaling=2^0
  "   1" : Constant  Value=1.001  OutDataType=sfix(16)  OutScaling=2^0
  "  1" : TransferFcn  Numerator=[5]  Denominator=[1/5 1]
  " 1" : Product  OutDataType=sfix(16)  OutScaling=2^0
  0.5 : Gain  Gain=0.5  ParameterDataType=sfix(16)  ParameterScaling=2^0  OutDataType=sfix(16)  OutScaling=2^0
  Abs : Abs
  Abs1 : Abs
  Demux2 : Demux  Outputs=2
  Mem : Memory
  Mem1 : Memory
  Relay : Relay  OnSwitchValue=0.5  OffSwitchValue=0.5  OutDataType=sfix(16)  OutScaling=2^0
  Relay1 : Relay  OnSwitchValue=0.5  OffSwitchValue=0.5  OutDataType=sfix(16)  OutScaling=2^0
  Sign : Signum
  Sign1 : Signum
  Sum : Sum  Inputs=|+-  OutDataType=sfix(16)  OutScaling=2^0
  Sum1 : Sum  Inputs=|+-  OutDataType=sfix(16)  OutScaling=2^0
  Sum3 : Sum  Inputs=++|  OutDataType=sfix(16)  OutScaling=2^0
  O1 : Outport  OutDataType=sfix(16)  OutScaling=2^0
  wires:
  0.5/1 -> O1/1
  Sum3/1 -> 0.5/1
  In1/1 -> Demux2/1
  Demux2/1 -> " "/1
  Demux2/2 -> " 1"/1
  " 1"/1 -> Sum1/1
  "   1"/1 -> " 1"/2
  Sum1/1 -> "  1"/1
  "  1"/1 -> Abs1/1, Sign1/1
  Abs1/1 -> Relay1/1
  Relay1/1 -> "    1"/1
  Sign1/1 -> "    1"/2
  Mem1/1 -> Sum1/2
  "    1"/1 -> Sum3/2, Mem1/1
  " "/1 -> Sum/1
  "   "/1 -> " "/2
  Sum/1 -> "  "/1
  "  "/1 -> Abs/1, Sign/1
  Abs/1 -> Relay/1
  Relay/1 -> "    "/1
  Sign/1 -> "    "/2
  Mem/1 -> Sum/2
  "    "/1 -> Sum3/1, Mem/1

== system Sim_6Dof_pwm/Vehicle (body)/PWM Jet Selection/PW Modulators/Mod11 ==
  In1 : Inport  OutDataType=sfix(16)  OutScaling=2^0
  " " : Product  OutDataType=sfix(16)  OutScaling=2^0
  "  " : TransferFcn  Numerator=[5]  Denominator=[1/5 1]
  "   " : Constant  Value=1.001  OutDataType=sfix(16)  OutScaling=2^0
  "    " : Product  OutDataType=sfix(16)  OutScaling=2^0
  "    1" : Product  OutDataType=sfix(16)  OutScaling=2^0
  "   1" : Constant  Value=1.001  OutDataType=sfix(16)  OutScaling=2^0
  "  1" : TransferFcn  Numerator=[5]  Denominator=[1/5 1]
  " 1" : Product  OutDataType=sfix(16)  OutScaling=2^0
  0.5 : Gain  Gain=0.5  ParameterDataType=sfix(16)  ParameterScaling=2^0  OutDataType=sfix(16)  OutScaling=2^0
  Abs : Abs
  Abs1 : Abs
  Demux2 : Demux  Outputs=2
  Mem : Memory
  Mem1 : Memory
  Relay : Relay  OnSwitchValue=0.5  OffSwitchValue=0.5  OutDataType=sfix(16)  OutScaling=2^0
  Relay1 : Relay  OnSwitchValue=0.5  OffSwitchValue=0.5  OutDataType=sfix(16)  OutScaling=2^0
  Sign : Signum
  Sign1 : Signum
  Sum : Sum  Inputs=|+-  OutDataType=sfix(16)  OutScaling=2^0
  Sum1 : Sum  Inputs=|+-  OutDataType=sfix(16)  OutScaling=2^0
  Sum3 : Sum  Inputs=++|  OutDataType=sfix(16)  OutScaling=2^0
  O1 : Outport  OutDataType=sfix(16)  OutScaling=2^0
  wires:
  0.5/1 -> O1/1
  Sum3/1 -> 0.5/1
  In1/1 -> Demux2/1
  Demux2/1 -> " "/1
  Demux2/2 -> " 1"/1
  " 1"/1 -> Sum1/1
  "   1"/1 -> " 1"/2
  Sum1/1 -> "  1"/1
  "  1"/1 -> Abs1/1, Sign1/1
  Abs1/1 -> Relay1/1
  Relay1/1 -> "    1"/1
  Sign1/1 -> "    1"/2
  Mem1/1 -> Sum1/2
  "    1"/1 -> Sum3/2, Mem1/1
  " "/1 -> Sum/1
  "   "/1 -> " "/2
  Sum/1 -> "  "/1
  "  "/1 -> Abs/1, Sign/1
  Abs/1 -> Relay/1
  Relay/1 -> "    "/1
  Sign/1 -> "    "/2
  Mem/1 -> Sum/2
  "    "/1 -> Sum3/1, Mem/1

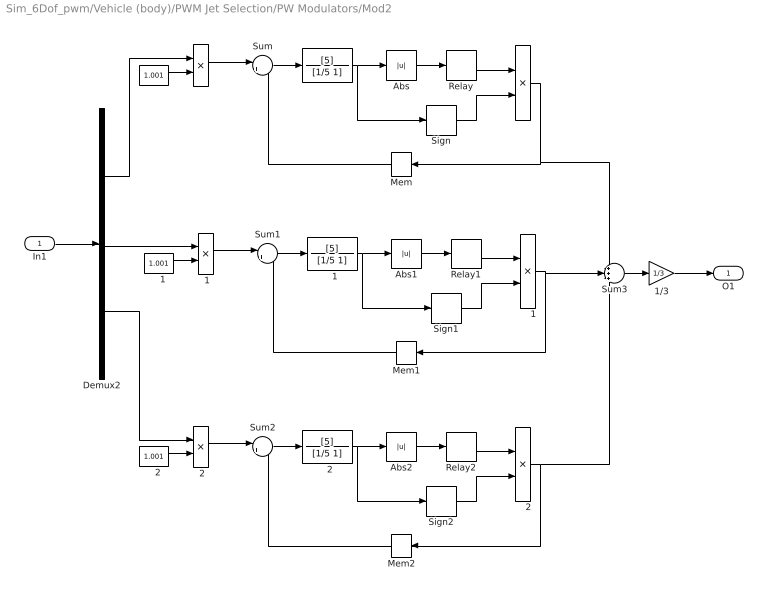
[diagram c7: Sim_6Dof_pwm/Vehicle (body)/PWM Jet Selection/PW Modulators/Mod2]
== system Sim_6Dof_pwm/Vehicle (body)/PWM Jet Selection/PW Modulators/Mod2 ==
  In1 : Inport  OutDataType=sfix(16)  OutScaling=2^0
  " " : Product  OutDataType=sfix(16)  OutScaling=2^0
  "  " : TransferFcn  Numerator=[5]  Denominator=[1/5 1]
  "   " : Constant  Value=1.001  OutDataType=sfix(16)  OutScaling=2^0
  "    " : Product  OutDataType=sfix(16)  OutScaling=2^0
  "    1" : Product  OutDataType=sfix(16)  OutScaling=2^0
  "    2" : Product  OutDataType=sfix(16)  OutScaling=2^0
  "   1" : Constant  Value=1.001  OutDataType=sfix(16)  OutScaling=2^0
  "   2" : Constant  Value=1.001  OutDataType=sfix(16)  OutScaling=2^0
  "  1" : TransferFcn  Numerator=[5]  Denominator=[1/5 1]
  "  2" : TransferFcn  Numerator=[5]  Denominator=[1/5 1]
  " 1" : Product  OutDataType=sfix(16)  OutScaling=2^0
  " 2" : Product  OutDataType=sfix(16)  OutScaling=2^0
  1/3 : Gain  Gain=1/3  ParameterDataType=sfix(16)  ParameterScaling=2^0  OutDataType=sfix(16)  OutScaling=2^0
  Abs : Abs
  Abs1 : Abs
  Abs2 : Abs
  Demux2 : Demux  Outputs=3
  Mem : Memory
  Mem1 : Memory
  Mem2 : Memory
  Relay : Relay  OnSwitchValue=0.5  OffSwitchValue=0.5  OutDataType=sfix(16)  OutScaling=2^0
  Relay1 : Relay  OnSwitchValue=0.5  OffSwitchValue=0.5  OutDataType=sfix(16)  OutScaling=2^0
  Relay2 : Relay  OnSwitchValue=0.5  OffSwitchValue=0.5  OutDataType=sfix(16)  OutScaling=2^0
  Sign : Signum
  Sign1 : Signum
  Sign2 : Signum
  Sum : Sum  Inputs=|+-  OutDataType=sfix(16)  OutScaling=2^0
  Sum1 : Sum  Inputs=|+-  OutDataType=sfix(16)  OutScaling=2^0
  Sum2 : Sum  Inputs=|+-  OutDataType=sfix(16)  OutScaling=2^0
  Sum3 : Sum  Inputs=+++  OutDataType=sfix(16)  OutScaling=2^0
  O1 : Outport  OutDataType=sfix(16)  OutScaling=2^0
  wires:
  1/3/1 -> O1/1
  Sum3/1 -> 1/3/1
  In1/1 -> Demux2/1
  Demux2/3 -> " 2"/1
  Demux2/1 -> " "/1
  Demux2/2 -> " 1"/1
  " 2"/1 -> Sum2/1
  "   2"/1 -> " 2"/2
  Sum2/1 -> "  2"/1
  "  2"/1 -> Abs2/1, Sign2/1
  Abs2/1 -> Relay2/1
  Relay2/1 -> "    2"/1
  Sign2/1 -> "    2"/2
  Mem2/1 -> Sum2/2
  "    2"/1 -> Sum3/3, Mem2/1
  " 1"/1 -> Sum1/1
  "   1"/1 -> " 1"/2
  Sum1/1 -> "  1"/1
  "  1"/1 -> Abs1/1, Sign1/1
  Abs1/1 -> Relay1/1
  Relay1/1 -> "    1"/1
  Sign1/1 -> "    1"/2
  Mem1/1 -> Sum1/2
  "    1"/1 -> Sum3/2, Mem1/1
  " "/1 -> Sum/1
  "   "/1 -> " "/2
  Sum/1 -> "  "/1
  "  "/1 -> Abs/1, Sign/1
  Abs/1 -> Relay/1
  Relay/1 -> "    "/1
  Sign/1 -> "    "/2
  Mem/1 -> Sum/2
  "    "/1 -> Sum3/1, Mem/1

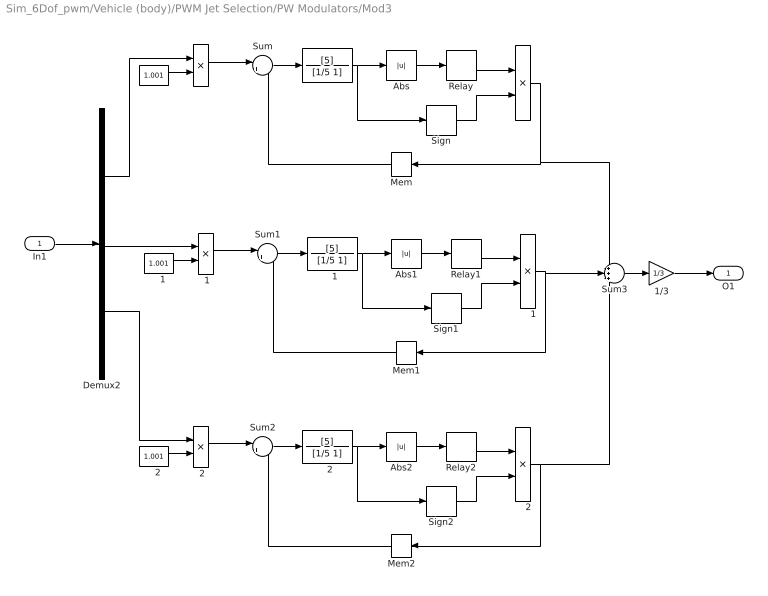
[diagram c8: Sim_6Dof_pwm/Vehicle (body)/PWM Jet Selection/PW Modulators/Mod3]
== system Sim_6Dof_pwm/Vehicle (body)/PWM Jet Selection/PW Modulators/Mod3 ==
  In1 : Inport  OutDataType=sfix(16)  OutScaling=2^0
  " " : Product  OutDataType=sfix(16)  OutScaling=2^0
  "  " : TransferFcn  Numerator=[5]  Denominator=[1/5 1]
  "   " : Constant  Value=1.001  OutDataType=sfix(16)  OutScaling=2^0
  "    " : Product  OutDataType=sfix(16)  OutScaling=2^0
  "    1" : Product  OutDataType=sfix(16)  OutScaling=2^0
  "    2" : Product  OutDataType=sfix(16)  OutScaling=2^0
  "   1" : Constant  Value=1.001  OutDataType=sfix(16)  OutScaling=2^0
  "   2" : Constant  Value=1.001  OutDataType=sfix(16)  OutScaling=2^0
  "  1" : TransferFcn  Numerator=[5]  Denominator=[1/5 1]
  "  2" : TransferFcn  Numerator=[5]  Denominator=[1/5 1]
  " 1" : Product  OutDataType=sfix(16)  OutScaling=2^0
  " 2" : Product  OutDataType=sfix(16)  OutScaling=2^0
  1/3 : Gain  Gain=1/3  ParameterDataType=sfix(16)  ParameterScaling=2^0  OutDataType=sfix(16)  OutScaling=2^0
  Abs : Abs
  Abs1 : Abs
  Abs2 : Abs
  Demux2 : Demux  Outputs=3
  Mem : Memory
  Mem1 : Memory
  Mem2 : Memory
  Relay : Relay  OnSwitchValue=0.5  OffSwitchValue=0.5  OutDataType=sfix(16)  OutScaling=2^0
  Relay1 : Relay  OnSwitchValue=0.5  OffSwitchValue=0.5  OutDataType=sfix(16)  OutScaling=2^0
  Relay2 : Relay  OnSwitchValue=0.5  OffSwitchValue=0.5  OutDataType=sfix(16)  OutScaling=2^0
  Sign : Signum
  Sign1 : Signum
  Sign2 : Signum
  Sum : Sum  Inputs=|+-  OutDataType=sfix(16)  OutScaling=2^0
  Sum1 : Sum  Inputs=|+-  OutDataType=sfix(16)  OutScaling=2^0
  Sum2 : Sum  Inputs=|+-  OutDataType=sfix(16)  OutScaling=2^0
  Sum3 : Sum  Inputs=+++  OutDataType=sfix(16)  OutScaling=2^0
  O1 : Outport  OutDataType=sfix(16)  OutScaling=2^0
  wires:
  1/3/1 -> O1/1
  Sum3/1 -> 1/3/1
  In1/1 -> Demux2/1
  Demux2/3 -> " 2"/1
  Demux2/1 -> " "/1
  Demux2/2 -> " 1"/1
  " 2"/1 -> Sum2/1
  "   2"/1 -> " 2"/2
  Sum2/1 -> "  2"/1
  "  2"/1 -> Abs2/1, Sign2/1
  Abs2/1 -> Relay2/1
  Relay2/1 -> "    2"/1
  Sign2/1 -> "    2"/2
  Mem2/1 -> Sum2/2
  "    2"/1 -> Sum3/3, Mem2/1
  " 1"/1 -> Sum1/1
  "   1"/1 -> " 1"/2
  Sum1/1 -> "  1"/1
  "  1"/1 -> Abs1/1, Sign1/1
  Abs1/1 -> Relay1/1
  Relay1/1 -> "    1"/1
  Sign1/1 -> "    1"/2
  Mem1/1 -> Sum1/2
  "    1"/1 -> Sum3/2, Mem1/1
  " "/1 -> Sum/1
  "   "/1 -> " "/2
  Sum/1 -> "  "/1
  "  "/1 -> Abs/1, Sign/1
  Abs/1 -> Relay/1
  Relay/1 -> "    "/1
  Sign/1 -> "    "/2
  Mem/1 -> Sum/2
  "    "/1 -> Sum3/1, Mem/1

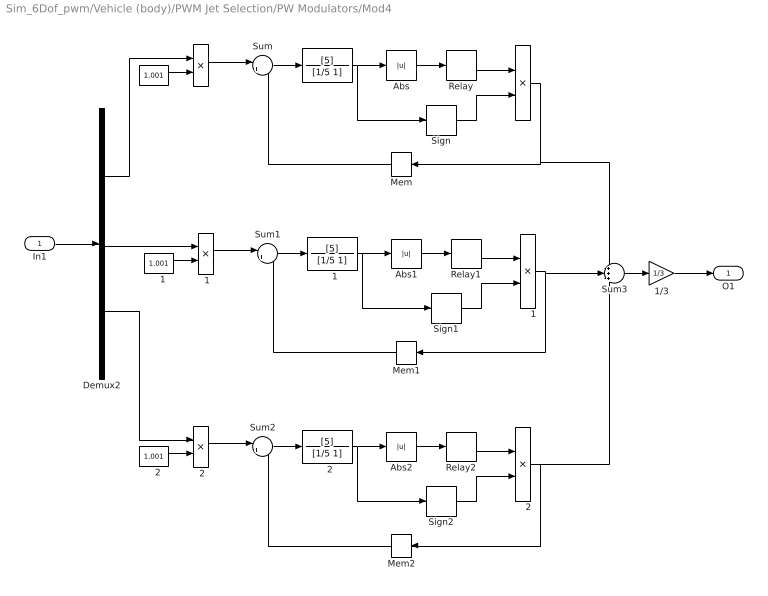
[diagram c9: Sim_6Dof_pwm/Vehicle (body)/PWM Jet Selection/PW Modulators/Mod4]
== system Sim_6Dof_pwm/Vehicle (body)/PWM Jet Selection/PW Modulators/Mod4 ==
  In1 : Inport  OutDataType=sfix(16)  OutScaling=2^0
  " " : Product  OutDataType=sfix(16)  OutScaling=2^0
  "  " : TransferFcn  Numerator=[5]  Denominator=[1/5 1]
  "   " : Constant  Value=1.001  OutDataType=sfix(16)  OutScaling=2^0
  "    " : Product  OutDataType=sfix(16)  OutScaling=2^0
  "    1" : Product  OutDataType=sfix(16)  OutScaling=2^0
  "    2" : Product  OutDataType=sfix(16)  OutScaling=2^0
  "   1" : Constant  Value=1.001  OutDataType=sfix(16)  OutScaling=2^0
  "   2" : Constant  Value=1.001  OutDataType=sfix(16)  OutScaling=2^0
  "  1" : TransferFcn  Numerator=[5]  Denominator=[1/5 1]
  "  2" : TransferFcn  Numerator=[5]  Denominator=[1/5 1]
  " 1" : Product  OutDataType=sfix(16)  OutScaling=2^0
  " 2" : Product  OutDataType=sfix(16)  OutScaling=2^0
  1/3 : Gain  Gain=1/3  ParameterDataType=sfix(16)  ParameterScaling=2^0  OutDataType=sfix(16)  OutScaling=2^0
  Abs : Abs
  Abs1 : Abs
  Abs2 : Abs
  Demux2 : Demux  Outputs=3
  Mem : Memory
  Mem1 : Memory
  Mem2 : Memory
  Relay : Relay  OnSwitchValue=0.5  OffSwitchValue=0.5  OutDataType=sfix(16)  OutScaling=2^0
  Relay1 : Relay  OnSwitchValue=0.5  OffSwitchValue=0.5  OutDataType=sfix(16)  OutScaling=2^0
  Relay2 : Relay  OnSwitchValue=0.5  OffSwitchValue=0.5  OutDataType=sfix(16)  OutScaling=2^0
  Sign : Signum
  Sign1 : Signum
  Sign2 : Signum
  Sum : Sum  Inputs=|+-  OutDataType=sfix(16)  OutScaling=2^0
  Sum1 : Sum  Inputs=|+-  OutDataType=sfix(16)  OutScaling=2^0
  Sum2 : Sum  Inputs=|+-  OutDataType=sfix(16)  OutScaling=2^0
  Sum3 : Sum  Inputs=+++  OutDataType=sfix(16)  OutScaling=2^0
  O1 : Outport  OutDataType=sfix(16)  OutScaling=2^0
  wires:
  1/3/1 -> O1/1
  Sum3/1 -> 1/3/1
  In1/1 -> Demux2/1
  Demux2/3 -> " 2"/1
  Demux2/1 -> " "/1
  Demux2/2 -> " 1"/1
  " 2"/1 -> Sum2/1
  "   2"/1 -> " 2"/2
  Sum2/1 -> "  2"/1
  "  2"/1 -> Abs2/1, Sign2/1
  Abs2/1 -> Relay2/1
  Relay2/1 -> "    2"/1
  Sign2/1 -> "    2"/2
  Mem2/1 -> Sum2/2
  "    2"/1 -> Sum3/3, Mem2/1
  " 1"/1 -> Sum1/1
  "   1"/1 -> " 1"/2
  Sum1/1 -> "  1"/1
  "  1"/1 -> Abs1/1, Sign1/1
  Abs1/1 -> Relay1/1
  Relay1/1 -> "    1"/1
  Sign1/1 -> "    1"/2
  Mem1/1 -> Sum1/2
  "    1"/1 -> Sum3/2, Mem1/1
  " "/1 -> Sum/1
  "   "/1 -> " "/2
  Sum/1 -> "  "/1
  "  "/1 -> Abs/1, Sign/1
  Abs/1 -> Relay/1
  Relay/1 -> "    "/1
  Sign/1 -> "    "/2
  Mem/1 -> Sum/2
  "    "/1 -> Sum3/1, Mem/1

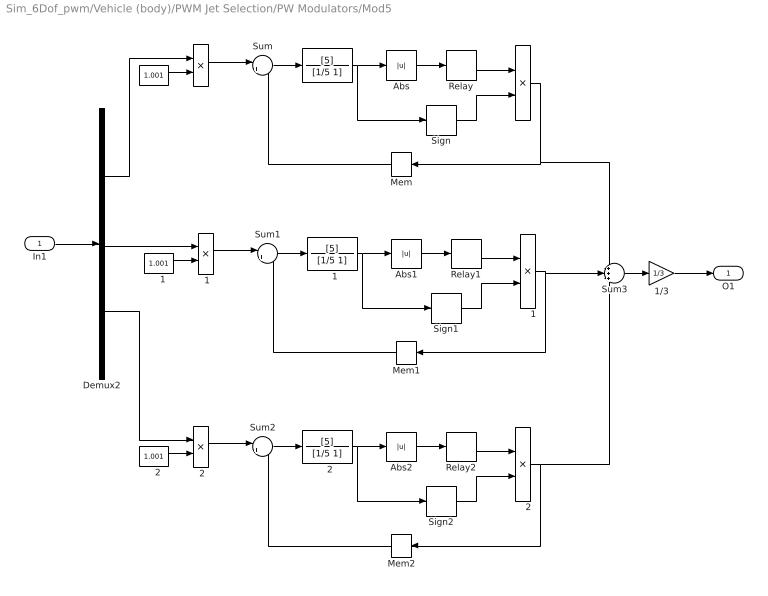
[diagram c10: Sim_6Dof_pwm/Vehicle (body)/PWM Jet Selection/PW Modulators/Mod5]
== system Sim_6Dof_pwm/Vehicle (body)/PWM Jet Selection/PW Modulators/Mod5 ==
  In1 : Inport  OutDataType=sfix(16)  OutScaling=2^0
  " " : Product  OutDataType=sfix(16)  OutScaling=2^0
  "  " : TransferFcn  Numerator=[5]  Denominator=[1/5 1]
  "   " : Constant  Value=1.001  OutDataType=sfix(16)  OutScaling=2^0
  "    " : Product  OutDataType=sfix(16)  OutScaling=2^0
  "    1" : Product  OutDataType=sfix(16)  OutScaling=2^0
  "    2" : Product  OutDataType=sfix(16)  OutScaling=2^0
  "   1" : Constant  Value=1.001  OutDataType=sfix(16)  OutScaling=2^0
  "   2" : Constant  Value=1.001  OutDataType=sfix(16)  OutScaling=2^0
  "  1" : TransferFcn  Numerator=[5]  Denominator=[1/5 1]
  "  2" : TransferFcn  Numerator=[5]  Denominator=[1/5 1]
  " 1" : Product  OutDataType=sfix(16)  OutScaling=2^0
  " 2" : Product  OutDataType=sfix(16)  OutScaling=2^0
  1/3 : Gain  Gain=1/3  ParameterDataType=sfix(16)  ParameterScaling=2^0  OutDataType=sfix(16)  OutScaling=2^0
  Abs : Abs
  Abs1 : Abs
  Abs2 : Abs
  Demux2 : Demux  Outputs=3
  Mem : Memory
  Mem1 : Memory
  Mem2 : Memory
  Relay : Relay  OnSwitchValue=0.5  OffSwitchValue=0.5  OutDataType=sfix(16)  OutScaling=2^0
  Relay1 : Relay  OnSwitchValue=0.5  OffSwitchValue=0.5  OutDataType=sfix(16)  OutScaling=2^0
  Relay2 : Relay  OnSwitchValue=0.5  OffSwitchValue=0.5  OutDataType=sfix(16)  OutScaling=2^0
  Sign : Signum
  Sign1 : Signum
  Sign2 : Signum
  Sum : Sum  Inputs=|+-  OutDataType=sfix(16)  OutScaling=2^0
  Sum1 : Sum  Inputs=|+-  OutDataType=sfix(16)  OutScaling=2^0
  Sum2 : Sum  Inputs=|+-  OutDataType=sfix(16)  OutScaling=2^0
  Sum3 : Sum  Inputs=+++  OutDataType=sfix(16)  OutScaling=2^0
  O1 : Outport  OutDataType=sfix(16)  OutScaling=2^0
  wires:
  1/3/1 -> O1/1
  Sum3/1 -> 1/3/1
  In1/1 -> Demux2/1
  Demux2/3 -> " 2"/1
  Demux2/1 -> " "/1
  Demux2/2 -> " 1"/1
  " 2"/1 -> Sum2/1
  "   2"/1 -> " 2"/2
  Sum2/1 -> "  2"/1
  "  2"/1 -> Abs2/1, Sign2/1
  Abs2/1 -> Relay2/1
  Relay2/1 -> "    2"/1
  Sign2/1 -> "    2"/2
  Mem2/1 -> Sum2/2
  "    2"/1 -> Sum3/3, Mem2/1
  " 1"/1 -> Sum1/1
  "   1"/1 -> " 1"/2
  Sum1/1 -> "  1"/1
  "  1"/1 -> Abs1/1, Sign1/1
  Abs1/1 -> Relay1/1
  Relay1/1 -> "    1"/1
  Sign1/1 -> "    1"/2
  Mem1/1 -> Sum1/2
  "    1"/1 -> Sum3/2, Mem1/1
  " "/1 -> Sum/1
  "   "/1 -> " "/2
  Sum/1 -> "  "/1
  "  "/1 -> Abs/1, Sign/1
  Abs/1 -> Relay/1
  Relay/1 -> "    "/1
  Sign/1 -> "    "/2
  Mem/1 -> Sum/2
  "    "/1 -> Sum3/1, Mem/1

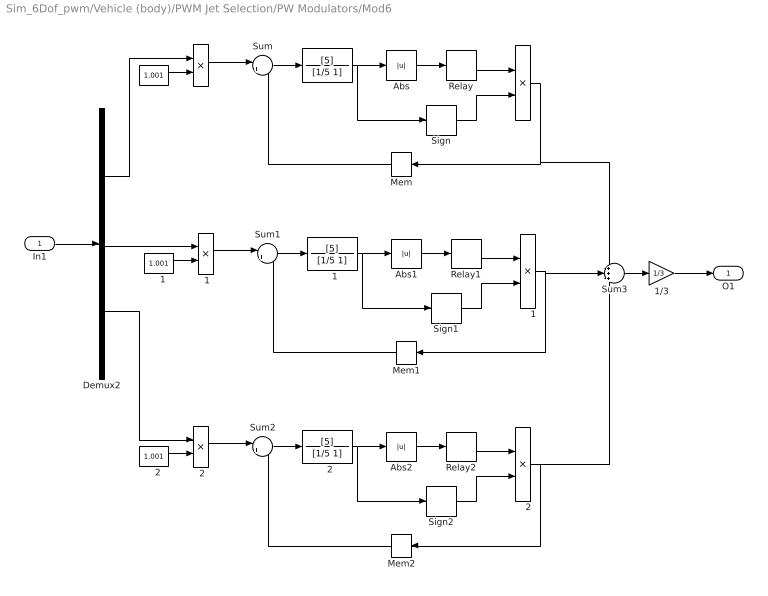
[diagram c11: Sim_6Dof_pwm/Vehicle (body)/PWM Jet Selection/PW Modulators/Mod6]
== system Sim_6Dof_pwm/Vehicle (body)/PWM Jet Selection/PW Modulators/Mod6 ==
  In1 : Inport  OutDataType=sfix(16)  OutScaling=2^0
  " " : Product  OutDataType=sfix(16)  OutScaling=2^0
  "  " : TransferFcn  Numerator=[5]  Denominator=[1/5 1]
  "   " : Constant  Value=1.001  OutDataType=sfix(16)  OutScaling=2^0
  "    " : Product  OutDataType=sfix(16)  OutScaling=2^0
  "    1" : Product  OutDataType=sfix(16)  OutScaling=2^0
  "    2" : Product  OutDataType=sfix(16)  OutScaling=2^0
  "   1" : Constant  Value=1.001  OutDataType=sfix(16)  OutScaling=2^0
  "   2" : Constant  Value=1.001  OutDataType=sfix(16)  OutScaling=2^0
  "  1" : TransferFcn  Numerator=[5]  Denominator=[1/5 1]
  "  2" : TransferFcn  Numerator=[5]  Denominator=[1/5 1]
  " 1" : Product  OutDataType=sfix(16)  OutScaling=2^0
  " 2" : Product  OutDataType=sfix(16)  OutScaling=2^0
  1/3 : Gain  Gain=1/3  ParameterDataType=sfix(16)  ParameterScaling=2^0  OutDataType=sfix(16)  OutScaling=2^0
  Abs : Abs
  Abs1 : Abs
  Abs2 : Abs
  Demux2 : Demux  Outputs=3
  Mem : Memory
  Mem1 : Memory
  Mem2 : Memory
  Relay : Relay  OnSwitchValue=0.5  OffSwitchValue=0.5  OutDataType=sfix(16)  OutScaling=2^0
  Relay1 : Relay  OnSwitchValue=0.5  OffSwitchValue=0.5  OutDataType=sfix(16)  OutScaling=2^0
  Relay2 : Relay  OnSwitchValue=0.5  OffSwitchValue=0.5  OutDataType=sfix(16)  OutScaling=2^0
  Sign : Signum
  Sign1 : Signum
  Sign2 : Signum
  Sum : Sum  Inputs=|+-  OutDataType=sfix(16)  OutScaling=2^0
  Sum1 : Sum  Inputs=|+-  OutDataType=sfix(16)  OutScaling=2^0
  Sum2 : Sum  Inputs=|+-  OutDataType=sfix(16)  OutScaling=2^0
  Sum3 : Sum  Inputs=+++  OutDataType=sfix(16)  OutScaling=2^0
  O1 : Outport  OutDataType=sfix(16)  OutScaling=2^0
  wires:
  1/3/1 -> O1/1
  Sum3/1 -> 1/3/1
  In1/1 -> Demux2/1
  Demux2/3 -> " 2"/1
  Demux2/1 -> " "/1
  Demux2/2 -> " 1"/1
  " 2"/1 -> Sum2/1
  "   2"/1 -> " 2"/2
  Sum2/1 -> "  2"/1
  "  2"/1 -> Abs2/1, Sign2/1
  Abs2/1 -> Relay2/1
  Relay2/1 -> "    2"/1
  Sign2/1 -> "    2"/2
  Mem2/1 -> Sum2/2
  "    2"/1 -> Sum3/3, Mem2/1
  " 1"/1 -> Sum1/1
  "   1"/1 -> " 1"/2
  Sum1/1 -> "  1"/1
  "  1"/1 -> Abs1/1, Sign1/1
  Abs1/1 -> Relay1/1
  Relay1/1 -> "    1"/1
  Sign1/1 -> "    1"/2
  Mem1/1 -> Sum1/2
  "    1"/1 -> Sum3/2, Mem1/1
  " "/1 -> Sum/1
  "   "/1 -> " "/2
  Sum/1 -> "  "/1
  "  "/1 -> Abs/1, Sign/1
  Abs/1 -> Relay/1
  Relay/1 -> "    "/1
  Sign/1 -> "    "/2
  Mem/1 -> Sum/2
  "    "/1 -> Sum3/1, Mem/1

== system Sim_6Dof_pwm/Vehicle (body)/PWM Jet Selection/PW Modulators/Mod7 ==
  In1 : Inport  OutDataType=sfix(16)  OutScaling=2^0
  " " : Product  OutDataType=sfix(16)  OutScaling=2^0
  "  " : TransferFcn  Numerator=[5]  Denominator=[1/5 1]
  "   " : Constant  Value=1.001  OutDataType=sfix(16)  OutScaling=2^0
  "    " : Product  OutDataType=sfix(16)  OutScaling=2^0
  "    1" : Product  OutDataType=sfix(16)  OutScaling=2^0
  "   1" : Constant  Value=1.001  OutDataType=sfix(16)  OutScaling=2^0
  "  1" : TransferFcn  Numerator=[5]  Denominator=[1/5 1]
  " 1" : Product  OutDataType=sfix(16)  OutScaling=2^0
  0.5 : Gain  Gain=0.5  ParameterDataType=sfix(16)  ParameterScaling=2^0  OutDataType=sfix(16)  OutScaling=2^0
  Abs : Abs
  Abs1 : Abs
  Demux2 : Demux  Outputs=2
  Mem : Memory
  Mem1 : Memory
  Relay : Relay  OnSwitchValue=0.5  OffSwitchValue=0.5  OutDataType=sfix(16)  OutScaling=2^0
  Relay1 : Relay  OnSwitchValue=0.5  OffSwitchValue=0.5  OutDataType=sfix(16)  OutScaling=2^0
  Sign : Signum
  Sign1 : Signum
  Sum : Sum  Inputs=|+-  OutDataType=sfix(16)  OutScaling=2^0
  Sum1 : Sum  Inputs=|+-  OutDataType=sfix(16)  OutScaling=2^0
  Sum3 : Sum  Inputs=++|  OutDataType=sfix(16)  OutScaling=2^0
  O1 : Outport  OutDataType=sfix(16)  OutScaling=2^0
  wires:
  0.5/1 -> O1/1
  Sum3/1 -> 0.5/1
  In1/1 -> Demux2/1
  Demux2/1 -> " "/1
  Demux2/2 -> " 1"/1
  " 1"/1 -> Sum1/1
  "   1"/1 -> " 1"/2
  Sum1/1 -> "  1"/1
  "  1"/1 -> Abs1/1, Sign1/1
  Abs1/1 -> Relay1/1
  Relay1/1 -> "    1"/1
  Sign1/1 -> "    1"/2
  Mem1/1 -> Sum1/2
  "    1"/1 -> Sum3/2, Mem1/1
  " "/1 -> Sum/1
  "   "/1 -> " "/2
  Sum/1 -> "  "/1
  "  "/1 -> Abs/1, Sign/1
  Abs/1 -> Relay/1
  Relay/1 -> "    "/1
  Sign/1 -> "    "/2
  Mem/1 -> Sum/2
  "    "/1 -> Sum3/1, Mem/1
